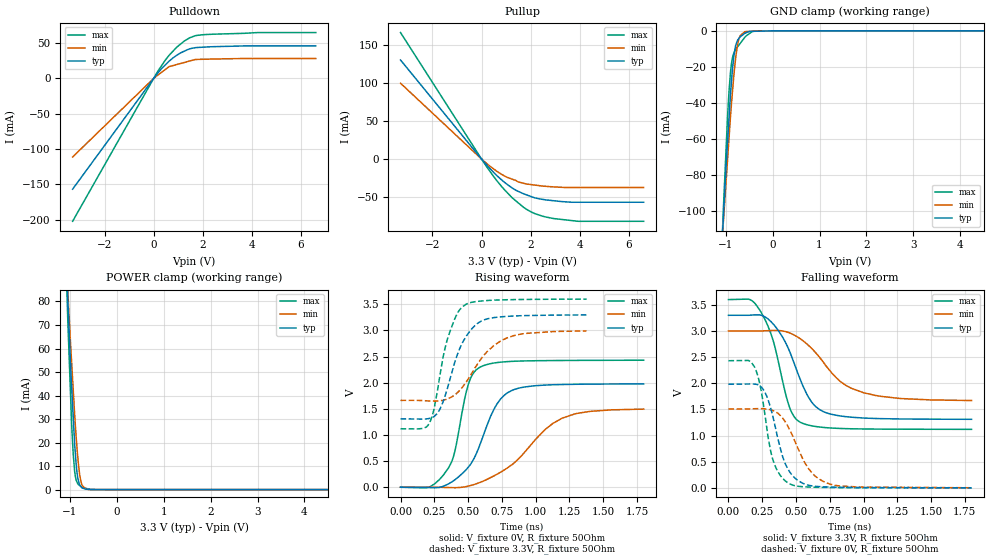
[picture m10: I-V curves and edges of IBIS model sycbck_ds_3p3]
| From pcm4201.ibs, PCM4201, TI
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|   sycbck_ds_3p3 Model
[Model]   sycbck_ds_3p3
Model_type   I/O
Polarity   Non-Inverting
Enable   Active-Low
Vinl = 0.99
Vinh = 2.31
Vmeas = 1.65
Vref = 1.65
Cref = 2pF
Rref = 50
|   typ   min   max
|   (nom PVT)   (fast PVT)   (slow PVT)
|C_comp from frequency sweep method (F=6.94MHz)
|Average
C_comp   1.209e-12   1.069e-12   1.381e-12
|ON state : BUFFER OUTPUT TURNED HIGH
|C_comp   1.247e-12   1.127e-12   1.445e-12
|OFF state: BUFFER IN HIGH IMPEDANCE
|C_comp   1.171e-12   1.010e-12   1.317e-12
|C_comp from LC tank measurement(L=1nH)
|Average
|Resonant Frequency(Hz)   7.760e+09   7.900e+09   7.495e+09
|C_comp   4.211e-13   4.066e-13   4.514e-13
|ON state : BUFFER OUTPUT TURNED HIGH
|Resonant Frequency(Hz)   7.720e+09   7.770e+09   7.490e+09
|C_comp   4.254e-13   4.200e-13   4.520e-13
|OFF state: BUFFER IN HIGH IMPEDANCE
|Resonant Frequency(Hz)   7.800e+09   8.030e+09   7.500e+09
|C_comp   4.168e-13   3.932e-13   4.508e-13
| Where nom  PVT is Nominal Process, 3.3V, 35C
|   Fast PVT is Strong Process,  3.6V, -10C
|   Slow PVT is Weak Process,   3V, 80C
[Model Spec]
Vinl   0.99   0.9   1.08
Vinh   2.31   2.1   2.52
[Voltage Range]   3.3   3   3.6
|Ambient Temperature   25   70   -10
|Junction Temperature
[Temperature Range]   35   80   -10
[Pullup Reference]   3.3   3   3.6
[Pulldown Reference]   0   0   0
[Power Clamp Reference]   3.3   3   3.6
[GND Clamp Reference]   0   0   0
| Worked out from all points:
|   slope of the pulldown table from 0 to 0.495 V, typ, clamps not added: 25 ohm
|   slope of the pullup table from 0 to 0.495 V, typ, clamps not added: 28.1 ohm
|   GND clamp passes 1 mA (typ) near -0.56 V on its own axis
|   POWER clamp passes 1 mA (typ) near -0.75 V on its own axis
|   falling waveform, V_fixture 3.3V, R_fixture 50Ohm: 20-80 % time 203ps typ, 298ps min, 152ps max; typ from 3.3 V to 1.31 V
|   rising waveform, V_fixture 0V, R_fixture 50Ohm: 20-80 % time 206ps typ, 367ps min, 121ps max; typ from 0 V to 1.98 V
|   rising waveform, V_fixture 3.3V, R_fixture 50Ohm: 20-80 % time 164ps typ, 237ps min, 127ps max; typ from 1.31 V to 3.3 V
|   falling waveform, V_fixture 0V, R_fixture 50Ohm: 20-80 % time 127ps typ, 180ps min, 101ps max; typ from 1.98 V to 0.002 V
[Pulldown]
|   Voltage   I(typ)   I(min)   I(max)
-3.3V     -156.9mA   -111.3mA   -202.4mA
18mV      811.1uA    603.1uA    1.128mA
172.8mV   7.787mA    4.701mA    10.34mA
633mV     24.59mA    16.74mA    32.89mA
939.6mV   32.82mA    19.66mA    44.25mA
1.246V    38.58mA    22.58mA    52.93mA
1.469V    41.87mA    24.7mA     57.59mA
1.692V    43.49mA    26.82mA    60.46mA
2.012V    44.26mA    27.15mA    61.95mA
4.208V    46.06mA    28.16mA    64.93mA
6.6V      46.06mA    28.16mA    64.97mA
[GND Clamp]
|   Voltage   I(typ)   I(min)   I(max)
-3.3V     -1.347A    -1.084A    -1.74A
-1.105V   -131.4mA   -127.7mA   -135mA
-1.051V   -104.8mA   -106.8mA   -100.1mA
-957.6mV  -60.85mA   -70.73mA   -46.53mA
-928.8mV  -48.57mA   -59.64mA   -33.58mA
-874.8mV  -27.6mA    -40.04mA   -17.83mA
-821.7mV  -13.1mA    -23.71mA   -12.19mA
-747mV    -5.242mA   -7.776mA   -8.933mA
-693mV    -3.387mA   -2.784mA   -7.073mA
-594mV    -1.406mA   -492.9uA   -3.663mA
-133.2mV  -88.06uA   -151.6nA   -18.24nA
6.6V      0A         0A         0A
[Pullup]
|   Voltage   I(typ)   I(min)   I(max)
-3.3V     130.7mA    100.1mA    166.9mA
172.8mV   -6.598mA   -4.879mA   -8.507mA
633mV     -22.16mA   -16.42mA   -28.97mA
939.6mV   -30.84mA   -22.42mA   -40.79mA
1.399V    -41.23mA   -28.32mA   -55.25mA
1.492V    -42.61mA   -30.16mA   -57.77mA
1.706V    -45.8mA    -31.93mA   -63.61mA
2.167V    -51.22mA   -34.33mA   -71.98mA
2.934V    -54.99mA   -36.73mA   -78.49mA
3.935V    -56.99mA   -37.53mA   -82.14mA
6.6V      -56.99mA   -37.53mA   -82.14mA
[POWER Clamp]
|   Voltage   I(typ)   I(min)   I(max)
-3.3V     1.329A     1.069A     1.72A
-1.086V   100.9mA    100.9mA    99.43mA
-1.044V   81.27mA    84.53mA    72.38mA
-961.2mV  43.68mA    53.95mA    27.77mA
-928.8mV  31.31mA    42.74mA    15.35mA
-896.4mV  19.07mA    31.56mA    7.563mA
-864.6mV  10.62mA    22.16mA    3.994mA
-831.6mV  5.062mA    13.97mA    2.491mA
-789mV    1.968mA    6.21mA     1.731mA
-745.8mV  785.2uA    2.283mA    1.149mA
-591mV    80.73uA    40.26uA    223.7uA
6.6V      0A         0A         0A
[Ramp]
R_load = 50
|   typ   min   max
dV/dt_r   1.18635/2.05648e-10   0.896791/3.65721e-10   1.45766/1.20551e-10
dV/dt_f   1.1931/2.02147e-10   0.797977/2.97255e-10   1.48806/1.51616e-10
[Falling Waveform]
V_fixture = 3.3V
V_fixture_min = 3V
V_fixture_max = 3.6V
R_fixture = 50Ohm
|   Time   V(typ)   V(min)   V(max)
0s        3.3V       3V         3.6V
159ps     3.302V     2.999V     3.601V
238.5ps   3.303V     3.001V     3.371V
334ps     3.125V     3.01V      2.79V
450.5ps   2.623V     2.965V     1.553V
529.5ps   2.086V     2.855V     1.258V
673.5ps   1.499V     2.5V       1.165V
830ps     1.375V     2.031V     1.136V
997ps     1.336V     1.822V     1.127V
1.8ns     1.312V     1.67V      1.12V
[Rising Waveform]
V_fixture = 0V
V_fixture_min = 0V
V_fixture_max = 0V
R_fixture = 50Ohm
|   Time   V(typ)   V(min)   V(max)
0s        738.5pV    1.224nV    535pV
214ps     -5.993mV   571.6uV    3.665mV
356ps     65.55mV    -5.948mV   373.1mV
402ps     141.8mV    -8.747mV   686.4mV
503ps     387.5mV    22.25mV    1.976V
590.5ps   833.9mV    94.44mV    2.3V
713ps     1.589V     247mV      2.384V
831ps     1.859V     443.6mV    2.408V
1.198ns   1.965V     1.322V     2.425V
1.8ns     1.977V     1.495V     2.429V
[Rising Waveform]
V_fixture = 3.3V
V_fixture_min = 3V
V_fixture_max = 3.6V
R_fixture = 50Ohm
|   Time   V(typ)   V(min)   V(max)
0s        1.308V     1.661V     1.118V
216.5ps   1.318V     1.65V      1.237V
251ps     1.358V     1.648V     1.535V
291ps     1.489V     1.654V     2.131V
344ps     1.864V     1.685V     2.806V
403.5ps   2.407V     1.77V      3.233V
462ps     2.783V     1.926V     3.459V
586ps     3.162V     2.418V     3.559V
786.5ps   3.267V     2.854V     3.586V
1.378ns   3.296V     2.991V     3.598V
[Falling Waveform]
V_fixture = 0V
V_fixture_min = 0V
V_fixture_max = 0V
R_fixture = 50Ohm
|   Time   V(typ)   V(min)   V(max)
0s        1.982V     1.508V     2.431V
192ps     1.986V     1.514V     2.317V
241.5ps   1.933V     1.515V     1.867V
296ps     1.665V     1.501V     936mV
327ps     1.381V     1.48V      556.3mV
400ps     607.6mV    1.339V     187.3mV
453ps     306.8mV    1.112V     78.62mV
596.5ps   48.6mV     356.2mV    16.73mV
747.5ps   16.26mV    75.78mV    7.717mV
1.8ns     1.876mV    2.915mV    1.173mV
